| IBIS file imxrt500_ewlb249_v1_3.ibs generated by Viper version: 2020.03.16
| This model valid for
| Part Numbers:   Temperature Range:   Package:
| MIMXRT533SFFOC/MRT533SFFOC   -20C~70C   FOWLP249
| MIMXRT533SFFOCR/MRT533SFFOC   -20C~70C   FOWLP249
| MIMXRT555SFFOC/MRT555SFFOC   -20C~70C   FOWLP249
| MIMXRT555SFFOCR/MRT555SFFOC   -20C~70C   FOWLP249
| MIMXRT595SFFOC/MRT595SFFOC   -20C~70C   FOWLP249
| MIMXRT595SFFOCR/MRT595SFFOC   -20C~70C   FOWLP249
[IBIS Ver]   5.0
[Comment Char]   |_char
[File Name]   imxrt500_ewlb249_v1_3.ibs
[File Rev]   1.2
[Date]   Wed Jan 20 13:06:18 2021
[Source]   NXP Viper 2020.03.16
[Notes]
   Warning 'pullup_ref' Exceeds 15 characters: MIPI_DSI_VDDHA18 was cut to MIPI_DSI_VDDHA1
   Warning 'pullup_ref' Exceeds 15 characters: MIPI_DSI_VDDA_CAP was cut to MIPI_DSI_VDDA_C
[Disclaimer] IMPORTANT NOTICE
  This information is provided on an AS IS basis and without warranty.
  IN NO EVENT SHALL NXP BE LIABLE FOR INCIDENTAL OR CONSEQUENTIAL
  DAMAGES ARISING FROM USE OF THIS INFORMATION. THIS DISCLAIMER OF
  WARRANTY EXTENDS TO THE USER OF THE INFORMATION, AND TO THEIR CUSTOMERS
  OR USERS OF PRODUCTS  AND IS IN LIEU OF ALL WARRANTIES WHETHER EXPRESS,
  IMPLIED, OR STATUTORY, INCLUDING IMPLIED WARRANTIES OF MERCHANTABILITY
  OR FITNESS FOR PARTICULAR PURPOSE.
  NXP does not represent or warrant that the information furnished
  hereunder is free of infringement of any third party patents,
  copyrights, trade secrets, or other intellectual property rights.
  NXP does not represent or warrant that the information is free of
  defect, or that it meets any particular standard, requirements or need
  of the user of the infomation or their customers.
  NXP reserves the right to change the information in this file
  without notice.
   http://www.nxp.com
[Copyright]   (C) Copyright NXP 2004 - 2021, All Rights Reserved.
|   BGA249
[Component]   BGA249
[Manufacturer]   NXP
[Package]
| variable   typ   min   max
R_pkg   0.15592   0.019296   0.4
L_pkg   9.605e-10   9.912e-11   2.758e-09
C_pkg   2.985e-13   9.631e-14   7.183e-13
[Pin] signal_name   model_name   R_pin   L_pin   C_pin
A1   GND   GND   NA   NA   NA
A2   XTALIN32KHZ   POWER   0.323   1.330e-09 4.451e-13
A4   XTALOUTSYS   POWER   0.23297   1.096e-09 4.846e-13
A6   PIO3_12   sd_mmc   0.14311   1.180e-09 3.826e-13
A8   PIO3_8   sd_mmc   0.12255   1.038e-09 3.823e-13
A10   PIO1_0   gpio   0.13766   1.041e-09 3.877e-13
A12   PIO0_28   gpio   0.16732   1.175e-09 4.245e-13
A14   PIO0_21   gpio   0.22629   1.768e-09 4.336e-13
A16   PIO0_16   gpio   0.23815   1.841e-09 4.605e-13
A17   GND   GND   NA   NA   NA
B1   MIPI_DSI_D0P   mipi   0.39132   1.963e-09 5.675e-13
B2   VDD_AO18   POWER   NA   NA   NA
B3   XTALOUT32KHZ   POWER   0.28473   1.432e-09 4.486e-13
B4   XTALINSYS   POWER   0.21088   9.995e-10 3.804e-13
B6   PIO3_18   sd_mmc   0.21102   1.406e-09 4.998e-13
B7   PIO3_13   sd_mmc   0.065009  4.534e-10 2.633e-13
B8   PIO3_9   sd_mmc   0.067056  5.910e-10 1.144e-13
B10   PIO2_29   gpio   0.13988   1.054e-09 2.088e-13
B11   PIO0_29   gpio   0.1449   1.036e-09 2.635e-13
B12   PIO0_14   gpio   0.21245   1.508e-09 4.307e-13
B14   PIO0_22   gpio   0.19354   1.505e-09 1.663e-13
B15   PIO0_15   gpio   0.19156   1.473e-09 2.499e-13
B16   PIO0_18   gpio   0.21271   1.627e-09 3.644e-13
B17   PIO0_17   gpio   0.2616   1.981e-09 4.581e-13
C2   MIPI_DSI_D0N   mipi   0.37397   1.899e-09 3.667e-13
C3   GND   GND   NA   NA   NA
C4   RESETN   gpio   0.13559   6.757e-10 3.401e-13
C5   LDO_ENABLE   gpio   0.032784  2.190e-10 2.165e-13
C6   PIO3_19   gpio   0.055897  5.682e-10 1.332e-13
C7   GND   GND   NA   NA   NA
C8   PIO3_10   sd_mmc   0.058396  5.217e-10 1.117e-13
C9   PIO3_16   sd_mmc   0.12717   1.005e-09 1.378e-13
C10   PIO3_11   sd_mmc   0.19256   1.616e-09 1.355e-13
C11   GND   GND   NA   NA   NA
C12   PIO0_25   gpio   0.12364   1.045e-09 1.356e-13
C13   PIO0_23   gpio   0.16274   1.396e-09 1.592e-13
C14   PIO2_31   gpio   0.16973   9.241e-10 3.844e-13
C15   GND   GND   NA   NA   NA
C16   PIO3_2   gpio   0.18067   1.120e-09 4.565e-13
D1   MIPI_DSI_CLKN   mipi   0.30826   1.261e-09 5.228e-13
D2   MIPI_DSI_CLKP   mipi   0.29277   1.248e-09 3.770e-13
D3   PMIC_MODE0   reset   0.085788  7.054e-10 2.084e-13
D4   VDDEAO   POWER   NA   NA   NA
D5   PMIC_IRQ   gpio   0.019296  9.912e-11 1.330e-13
D6   PIO3_20   gpio   0.12395   8.467e-10 1.799e-13
D7   VSS_ANA   GND   NA   NA   NA
D8   PIO3_17   sd_mmc   0.059128  2.748e-10 1.732e-13
D9   PIO3_14   sd_mmc   0.047493  2.375e-10 1.631e-13
D10   PIO2_30   gpio   0.069171  3.220e-10 1.808e-13
D11   VSS_ADC_ANA   GND   NA   NA   NA
D12   PIO0_31   gpio   0.21896   1.731e-09 2.097e-13
D13   PIO0_24   gpio   0.15029   1.266e-09 1.559e-13
D14   PIO0_30   gpio   0.10947   5.921e-10 2.238e-13
D15   PIO3_3   gpio   0.13521   8.908e-10 1.680e-13
D16   PIO3_1   gpio   0.11241   8.008e-10 2.775e-13
D17   PIO2_15   gpio   0.15691   1.163e-09 4.295e-13
E3   MIPI_DSI_D1P   mipi   0.22048   8.959e-10 4.982e-13
E4   PMIC_MODE1   reset   0.077495  3.186e-10 1.888e-13
E5   PIO3_21   gpio   0.24735   1.577e-09 3.754e-13
E6   VDD_PLL18   POWER   NA   NA   NA
E7   GND   GND   NA   NA   NA
E8   VDD_FUSE18   POWER   NA   NA   NA
E9   VDDE1   POWER   NA   NA   NA
E10   PIO3_15   sd_mmc   0.12196   5.270e-10 2.435e-13
E11   GND   GND   NA   NA   NA
E12   VDD33_ADC_ANA   POWER   NA   NA   NA
E13   PIO4_18   gpio   0.07626   3.382e-10 1.901e-13
E14   PIO0_12   gpio   0.022368  1.796e-10 1.296e-13
E15   PIO2_14   gpio   0.081977  7.304e-10 1.096e-13
F1   PIO4_14   sd_mmc   0.25944   1.688e-09 5.184e-13
F2   PIO4_17   sd_mmc   0.25835   1.776e-09 3.608e-13
F3   MIPI_DSI_D1N   mipi   0.21045   9.219e-10 3.502e-13
F4   MIPI_DSI_VSS   GND   NA   NA   NA
F5   MIPI_DSI_VDDA_CAP   POWER   NA   NA   NA
F6   VDDE4   POWER   NA   NA   NA
F7   VDDE4   POWER   NA   NA   NA
F8   MIPI_DSI_VDDHA18   POWER   NA   NA   NA
F9   VDDE1   POWER   NA   NA   NA
F10   VDDE1   POWER   NA   NA   NA
F11   VDDE1   POWER   NA   NA   NA
F12   VREFH_ANA18   POWER   NA   NA   NA
F13   PIO0_19   gpio   0.097275  4.356e-10 2.152e-13
F14   PIO0_0   gpio   0.088128  3.411e-10 1.672e-13
F15   PIO0_13   gpio   0.07821   6.497e-10 1.711e-13
F16   PIO0_5   gpio   0.081289  5.963e-10 2.780e-13
F17   PIO0_6   gpio   0.13882   1.098e-09 3.874e-13
G2   PIO4_13   sd_mmc   0.22197   1.542e-09 4.236e-13
G3   GND   GND   NA   NA   NA
G4   GND   GND   NA   NA   NA
G5   GND   GND   NA   NA   NA
G6   VDD1V8   POWER   NA   NA   NA
G7   GND   GND   NA   NA   NA
G8   GND   GND   NA   NA   NA
G9   VDDCORE_CAP   POWER   NA   NA   NA
G10   GND   GND   NA   NA   NA
G11   GND   GND   NA   NA   NA
G12   VREFL_ANA   POWER   NA   NA   NA
G13   GND   GND   NA   NA   NA
G14   GND   GND   NA   NA   NA
G15   GND   GND   NA   NA   NA
G16   PIO0_1   gpio   0.10247   4.579e-10 3.732e-13
H1   PIO4_12   sd_mmc   0.13261   1.127e-09 1.525e-13
H2   PIO4_11   sd_mmc   0.084302  6.153e-10 2.604e-13
H3   PIO4_16   sd_mmc   0.11951   1.103e-09 1.622e-13
H4   PIO5_16   sd_mmc   0.062756  3.311e-10 1.766e-13
H5   PIO5_15   sd_mmc   0.072627  3.073e-10 1.838e-13
H6   VDD18_IOREF_1   POWER   NA   NA   NA
H7   VDD1V8_DRV   POWER   NA   NA   NA
H8   VDDCORE_CAP   POWER   NA   NA   NA
H9   VDDCORE_CAP   POWER   NA   NA   NA
H10   VDDCORE_CAP   POWER   NA   NA   NA
H11   GND   GND   NA   NA   NA
H12   PIO0_8   gpio   0.12057   4.423e-10 2.342e-13
H13   VDD18_ADC_ANA   POWER   NA   NA   NA
H14   PIO0_4   gpio   0.047831  2.176e-10 1.585e-13
H15   PIO0_3   gpio   0.058566  4.883e-10 1.263e-13
H16   PIO0_2   gpio   0.092167  5.766e-10 3.745e-13
H17   PIO0_9   gpio   0.14943   8.879e-10 4.225e-13
J3   PIO5_17   sd_mmc   0.038017  3.866e-10 9.631e-14
J4   PIO5_18   sd_mmc   0.073931  3.262e-10 1.803e-13
J5   VDDE1   POWER   NA   NA   NA
J6   VDDE1   POWER   NA   NA   NA
J7   VDD1V8_DRV   POWER   NA   NA   NA
J8   MIPI_DSI_VDD11   POWER   NA   NA   NA
J9   VDDCORE_CAP   POWER   NA   NA   NA
J10   VDDCORE_CAP   POWER   NA   NA   NA
J11   VDDCORE_CAP   POWER   NA   NA   NA
J12   VDDE0   POWER   NA   NA   NA
J13   VDDE0   POWER   NA   NA   NA
J14   VDD18_IOREF_0   POWER   NA   NA   NA
J15   PIO0_7   gpio   0.062602  5.461e-10 1.030e-13
K1   PIO1_4   gpio   0.12726   1.026e-09 4.289e-13
K2   PIO1_3   gpio   0.064288  5.590e-10 3.224e-13
K3   PIO4_15   sd_mmc   0.052393  4.047e-10 1.440e-13
K4   PMIC_I2C_SCL   gpio   0.041685  2.210e-10 1.504e-13
K5   VDD_USB33   POWER   NA   NA   NA
K6   PMIC_I2C_SDA   gpio   0.13049   4.317e-10 3.502e-13
K7   GND   GND   NA   NA   NA
K8   VDDCORE_CAP   POWER   NA   NA   NA
K9   VDDCORE_CAP   POWER   NA   NA   NA
K10   VDDCORE_CAP   POWER   NA   NA   NA
K11   GND   GND   NA   NA   NA
K12   VDDE0   POWER   NA   NA   NA
K13   PIO1_11   gpio   0.073705  2.916e-10 3.894e-13
K14   PIO1_12   gpio   0.050827  2.077e-10 1.709e-13
K15   PIO0_11   gpio   0.061973  4.783e-10 2.714e-13
K16   PIO0_10   gpio   0.12779   7.528e-10 3.663e-13
K17   PIO1_13   gpio   0.13572   9.556e-10 4.001e-13
L2   PIO1_5   gpio   0.075752  5.651e-10 2.551e-13
L3   GND   GND   NA   NA   NA
L4   GND   GND   NA   NA   NA
L5   GND   GND   NA   NA   NA
L6   GND   GND   NA   NA   NA
L7   GND   GND   NA   NA   NA
L8   GND   GND   NA   NA   NA
L9   VDDCORE_CAP   POWER   NA   NA   NA
L10   GND   GND   NA   NA   NA
L11   GND   GND   NA   NA   NA
L12   GND   GND   NA   NA   NA
L13   GND   GND   NA   NA   NA
L14   GND   GND   NA   NA   NA
L15   GND   GND   NA   NA   NA
L16   PIO1_14   gpio   0.086255  5.497e-10 3.068e-13
M1   PIO1_7   gpio   0.19046   1.385e-09 5.761e-13
M2   PIO2_25   gpio   0.13329   1.029e-09 3.646e-13
M3   PIO2_27   gpio   0.082138  2.978e-10 1.572e-13
M4   PIO2_26   gpio   0.085997  3.288e-10 1.757e-13
M5   PIO1_10   gpio   0.079525  3.383e-10 1.749e-13
M6   VDD_USB18   POWER   NA   NA   NA
M7   GND   GND   NA   NA   NA
M8   VDDE3   POWER   NA   NA   NA
M9   PIO5_1   gpiohv   0.17413   6.089e-10 4.540e-13
M10   VDDE0   POWER   NA   NA   NA
M11   GND   GND   NA   NA   NA
M12   VDDE0   POWER   NA   NA   NA
M13   PIO3_29   gpio   0.20028   7.768e-10 3.196e-13
M14   PIO4_3   gpio   0.072546  3.197e-10 1.837e-13
M15   PIO4_1   gpio   0.11381   8.533e-10 2.816e-13
M16   PIO1_15   gpio   0.16285   5.641e-10 4.457e-13
M17   PIO4_2   gpio   0.15728   1.014e-09 4.269e-13
N3   PIO2_24   gpio   0.11438   5.537e-10 1.723e-13
N4   PIO1_6   gpio   0.062866  3.020e-10 1.892e-13
N5   PIO2_10   gpio   0.073482  3.155e-10 1.841e-13
N6   VDDE2   POWER   NA   NA   NA
N7   GND   GND   NA   NA   NA
N8   PIO4_30   gpiohv   0.11743   4.531e-10 2.355e-13
N9   VDDE3   POWER   NA   NA   NA
N10   PIO4_31   gpiohv   0.17786   6.915e-10 3.013e-13
N11   GND   GND   NA   NA   NA
N12   PIO1_24   sd_mmc   0.27515   9.660e-10 3.982e-13
N13   PIO3_28   gpio   0.18841   6.032e-10 2.830e-13
N14   PIO3_27   gpio   0.22419   7.513e-10 3.286e-13
N15   PIO4_0   gpio   0.050214  4.488e-10 9.853e-14
P1   PIO2_28   gpio   0.23077   8.666e-10 4.913e-13
P2   PIO5_4   gpio   0.18895   8.361e-10 2.819e-13
P3   PIO5_8   gpio   0.16805   5.890e-10 3.961e-13
P4   PIO2_7   sd_mmc   0.046303  2.501e-10 1.483e-13
P5   PIO2_5   sd_mmc   0.036306  2.135e-10 1.439e-13
P6   PIO2_4   sd_mmc   0.069851  3.058e-10 1.856e-13
P7   VDDE2   POWER   NA   NA   NA
P8   PIO4_29   gpiohv   0.074088  3.644e-10 1.958e-13
P9   PIO4_27   gpiohv   0.15417   6.758e-10 2.585e-13
P10   PIO4_21   gpiohv   0.1396   5.865e-10 2.562e-13
P11   GND   GND   NA   NA   NA
P12   PIO5_0   gpiohv   0.31252   2.244e-09 3.349e-13
P13   PIO1_27   sd_mmc   0.23594   1.837e-09 2.443e-13
P14   PIO1_26   sd_mmc   0.30392   1.154e-09 4.566e-13
P15   PIO4_6   gpio   0.061648  4.596e-10 1.742e-13
P16   PIO4_5   gpio   0.20809   1.756e-09 4.205e-13
P17   PIO4_4   gpio   0.1891   1.545e-09 3.954e-13
R2   PIO2_11   gpio   0.12089   8.885e-10 1.990e-13
R3   GND   GND   NA   NA   NA
R4   PIO2_6   sd_mmc   0.067012  6.136e-10 9.890e-14
R5   PIO1_30   sd_mmc   0.068108  3.900e-10 1.962e-13
R6   PIO1_31   sd_mmc   0.056674  4.622e-10 1.939e-13
R7   GND   GND   NA   NA   NA
R8   PIO4_20   gpiohv   0.057557  5.489e-10 1.040e-13
R9   PIO5_2   gpiohv   0.091773  6.332e-10 1.818e-13
R10   PIO5_3   gpiohv   0.13625   8.187e-10 2.283e-13
R11   GND   GND   NA   NA   NA
R12   PIO1_23   sd_mmc   0.30732   1.355e-09 4.114e-13
R13   PIO1_22   sd_mmc   0.2423   1.910e-09 2.292e-13
R14   PIO1_25   sd_mmc   0.3338   2.453e-09 2.757e-13
R15   GND   GND   NA   NA   NA
R16   PIO3_25   gpio   0.27408   1.989e-09 2.302e-13
T1   USB0_DM   usbdpdm   0.35276   1.717e-09 5.051e-13
T2   USB0_VBUS_DETECT   POWER   0.26142   1.418e-09 4.000e-13
T3   PIO2_9   gpio   0.092275  7.827e-10 3.446e-13
T4   PIO2_1   sd_mmc   0.083664  7.075e-10 3.423e-13
T6   PIO2_8   sd_mmc   0.11338   1.080e-09 2.706e-13
T7   PIO2_2   sd_mmc   0.11182   1.072e-09 2.535e-13
T8   PIO4_23   gpiohv   0.087906  6.854e-10 2.884e-13
T10   PIO4_24   gpiohv   0.13973   9.951e-10 2.208e-13
T11   PIO4_25   gpiohv   0.25374   1.734e-09 2.601e-13
T12   PIO4_26   gpiohv   0.26837   1.817e-09 2.982e-13
T14   PIO1_21   sd_mmc   0.36032   1.841e-09 4.475e-13
T15   PIO1_20   sd_mmc   0.38127   1.797e-09 4.826e-13
T16   PIO3_26   gpio   0.28345   1.995e-09 4.672e-13
T17   PIO1_18   sd_mmc   0.394   2.758e-09 5.564e-13
U1   GND   GND   NA   NA   NA
U2   USB0_DP   usbdpdm   0.33611   1.796e-09 4.815e-13
U4   PIO2_0   sd_mmc   0.18718   1.342e-09 4.224e-13
U6   PIO2_3   sd_mmc   0.17593   1.363e-09 5.005e-13
U8   PIO4_28   gpiohv   0.14778   1.113e-09 3.807e-13
U10   PIO4_22   gpiohv   0.19253   1.246e-09 4.489e-13
U12   PIO1_29   sd_mmc   0.28287   1.985e-09 5.064e-13
U14   PIO1_28   sd_mmc   0.29826   2.149e-09 5.288e-13
U16   PIO1_19   sd_mmc   0.4   2.303e-09 7.183e-13
U17   GND   GND   NA   NA   NA
[Pin Mapping]   pulldown_ref   pullup_ref
A1   GND   NC
A2   NC   VDDEAO
A4   NC   VDD_FUSE18
A6   GND   VDDE4
A8   GND   VDDE4
A10   GND   VDDE1
A12   GND   VDDE1
A14   GND   VDDE1
A16   GND   VDDE1
A17   GND   NC
B1   GND   MIPI_DSI_VDDHA1
B2   NC   VDD_AO18
B3   NC   VDDEAO
B4   NC   VDD_FUSE18
B6   GND   VDDE4
B7   GND   VDDE4
B8   GND   VDDE4
B10   GND   VDDE1
B11   GND   VDDE1
B12   GND   VDDE1
B14   GND   VDDE1
B15   GND   VDDE1
B16   GND   VDDE1
B17   GND   VDDE1
C2   GND   MIPI_DSI_VDDHA1
C3   GND   NC
C4   GND   VDDEAO
C5   GND   VDDEAO
C6   GND   VDDE4
C7   GND   NC
C8   GND   VDDE4
C9   GND   VDDE4
C10   GND   VDDE4
C11   GND   NC
C12   GND   VDDE1
C13   GND   VDDE1
C14   GND   VDDE1
C15   GND   NC
C16   GND   VDDE1
D1   GND   MIPI_DSI_VDDHA1
D2   GND   MIPI_DSI_VDDHA1
D3   GND   VDDEAO
D4   NC   VDDEAO
D5   GND   VDDEAO
D6   GND   VDDE4
D7   GND   NC
D8   GND   VDDE4
D9   GND   VDDE4
D10   GND   VDDE1
D11   VSS_ADC_ANA   NC
D12   GND   VDDE1
D13   GND   VDDE1
D14   GND   VDDE1
D15   GND   VDDE1
D16   GND   VDDE1
D17   GND   VDDE0
E3   GND   MIPI_DSI_VDDHA1
E4   GND   VDDEAO
E5   GND   VDDE4
E6   NC   VDD_PLL18
E7   GND   NC
E8   NC   VDD_FUSE18
E9   NC   VDDE1
E10   GND   VDDE4
E11   GND   NC
E12   NC   VDD33_ADC_ANA
E13   GND   VDDE1
E14   GND   VDDE0
E15   GND   VDDE0
F1   GND   VDDE1
F2   GND   VDDE1
F3   GND   MIPI_DSI_VDDHA1
F4   GND   NC
F5   NC   MIPI_DSI_VDDA_C
F6   NC   VDDE4
F7   NC   VDDE4
F8   NC   MIPI_DSI_VDDHA1
F9   NC   VDDE1
F10   NC   VDDE1
F11   NC   VDDE1
F12   NC   VDD18_ADC_ANA
F13   GND   VDDE1
F14   GND   VDDE0
F15   GND   VDDE0
F16   GND   VDDE0
F17   GND   VDDE0
G2   GND   VDDE1
G3   GND   NC
G4   GND   NC
G5   GND   NC
G6   NC   VDDEAO
G7   GND   NC
G8   GND   NC
G9   NC   VDDE0
G10   GND   NC
G11   GND   NC
G12   NC   VDD18_ADC_ANA
G13   GND   NC
G14   GND   NC
G15   GND   NC
G16   GND   VDDE0
H1   GND   VDDE1
H2   GND   VDDE1
H3   GND   VDDE1
H4   GND   VDDE1
H5   GND   VDDE1
H6   NC   VDDE1
H7   NC   VDDEAO
H8   NC   VDDE0
H9   NC   VDDE0
H10   NC   VDDE0
H11   GND   NC
H12   GND   VDDE0
H13   NC   VDD33_ADC_ANA
H14   GND   VDDE0
H15   GND   VDDE0
H16   GND   VDDE0
H17   GND   VDDE0
J3   GND   VDDE1
J4   GND   VDDE1
J5   NC   VDDE1
J6   NC   VDDE1
J7   NC   VDDEAO
J8   NC   MIPI_DSI_VDD11
J9   NC   VDDE0
J10   NC   VDDE0
J11   NC   VDDE0
J12   NC   VDDE0
J13   NC   VDDE0
J14   NC   VDDE0
J15   GND   VDDE0
K1   GND   VDDE1
K2   GND   VDDE1
K3   GND   VDDE1
K4   GND   VDDE1
K5   NC   VDD_USB33
K6   GND   VDDE1
K7   GND   NC
K8   NC   VDDE0
K9   NC   VDDE0
K10   NC   VDDE0
K11   GND   NC
K12   NC   VDDE0
K13   GND   VDDE0
K14   GND   VDDE0
K15   GND   VDDE0
K16   GND   VDDE0
K17   GND   VDDE0
L2   GND   VDDE1
L3   GND   NC
L4   GND   NC
L5   GND   NC
L6   GND   NC
L7   GND   NC
L8   GND   NC
L9   NC   VDDE0
L10   GND   NC
L11   GND   NC
L12   GND   NC
L13   GND   NC
L14   GND   NC
L15   GND   NC
L16   GND   VDDE0
M1   GND   VDDE1
M2   GND   VDDE1
M3   GND   VDDE1
M4   GND   VDDE1
M5   GND   VDDE1
M6   NC   VDD_USB33
M7   GND   NC
M8   NC   VDDE3
M9   GND   VDDE3
M10   NC   VDDE0
M11   GND   NC
M12   NC   VDDE0
M13   GND   VDDE0
M14   GND   VDDE0
M15   GND   VDDE0
M16   GND   VDDE0
M17   GND   VDDE0
N3   GND   VDDE1
N4   GND   VDDE1
N5   GND   VDDE2
N6   NC   VDDE2
N7   GND   NC
N8   GND   VDDE3
N9   NC   VDDE3
N10   GND   VDDE3
N11   GND   NC
N12   GND   VDDE0
N13   GND   VDDE0
N14   GND   VDDE0
N15   GND   VDDE0
P1   GND   VDDE1
P2   GND   VDDE1
P3   GND   VDDE1
P4   GND   VDDE2
P5   GND   VDDE2
P6   GND   VDDE2
P7   NC   VDDE2
P8   GND   VDDE3
P9   GND   VDDE3
P10   GND   VDDE3
P11   GND   NC
P12   GND   VDDE3
P13   GND   VDDE0
P14   GND   VDDE0
P15   GND   VDDE0
P16   GND   VDDE0
P17   GND   VDDE0
R2   GND   VDDE2
R3   GND   NC
R4   GND   VDDE2
R5   GND   VDDE2
R6   GND   VDDE2
R7   GND   NC
R8   GND   VDDE3
R9   GND   VDDE3
R10   GND   VDDE3
R11   GND   NC
R12   GND   VDDE0
R13   GND   VDDE0
R14   GND   VDDE0
R15   GND   NC
R16   GND   VDDE0
T1   GND   VDD_USB33
T2   NC   VDD_USB33
T3   GND   VDDE2
T4   GND   VDDE2
T6   GND   VDDE2
T7   GND   VDDE2
T8   GND   VDDE3
T10   GND   VDDE3
T11   GND   VDDE3
T12   GND   VDDE3
T14   GND   VDDE0
T15   GND   VDDE0
T16   GND   VDDE0
T17   GND   VDDE0
U1   GND   NC
U2   GND   VDD_USB33
U4   GND   VDDE2
U6   GND   VDDE2
U8   GND   VDDE3
U10   GND   VDDE3
U12   GND   VDDE0
U14   GND   VDDE0
U16   GND   VDDE0
U17   GND   NC
[Diff Pin]  inv_pin  vdiff  tdelay_typ tdelay_min tdelay_max
B1   C2   NA   NA   NA   NA
D2   D1   NA   NA   NA   NA
E3   F3   NA   NA   NA   NA
T1   U2   NA   NA   NA   NA
|*   Model Selector   *
[Model Selector] gpio
io_obe1dse0sre0_lr   5mA current driving capability, w/o slew rate (Low Range Typ: 1.80V, Min: 1.71V, Max: 1.98V)
io_obe1dse0sre1_lr   5mA current driving capability, with slew rate (Low Range Typ: 1.80V, Min: 1.71V, Max: 1.98V)
io_obe1dse1sre0_lr   10mA current driving capability, w/o slew rate (Low Range Typ: 1.80V, Min: 1.71V, Max: 1.98V)
io_obe1dse1sre1_lr   10mA current driving capability, with slew rate (Low Range Typ: 1.80V, Min: 1.71V, Max: 1.98V)
[Model Selector] gpiohv
io_obe1dse0sre0_hr   5mA current driving capability, w/o slew rate (High Range Typ: 3.30V, Min: 3.00V, Max: 3.60V)
io_obe1dse0sre0_lr   5mA current driving capability, w/o slew rate (Low Range Typ: 1.80V, Min: 1.71V, Max: 1.98V)
io_obe1dse0sre0_nr   5mA current driving capability, w/o slew rate (Cont. Range Typ: 3.30V, Min: 2.70V, Max: 3.60V)
io_obe1dse0sre1_hr   5mA current driving capability, with slew rate (High Range Typ: 3.30V, Min: 3.00V, Max: 3.60V)
io_obe1dse0sre1_lr   5mA current driving capability, with slew rate (Low Range Typ: 1.80V, Min: 1.71V, Max: 1.98V)
io_obe1dse0sre1_nr   5mA current driving capability, with slew rate (Cont. Range Typ: 3.30V, Min: 2.70V, Max: 3.60V)
io_obe1dse1sre0_hr   10mA current driving capability, w/o slew rate (High Range Typ: 3.30V, Min: 3.00V, Max: 3.60V)
io_obe1dse1sre0_lr   10mA current driving capability, w/o slew rate (Low Range Typ: 1.80V, Min: 1.71V, Max: 1.98V)
io_obe1dse1sre0_nr   10mA current driving capability, w/o slew rate (Cont. Range Typ: 3.30V, Min: 2.70V, Max: 3.60V)
io_obe1dse1sre1_hr   10mA current driving capability, with slew rate (High Range Typ: 3.30V, Min: 3.00V, Max: 3.60V)
io_obe1dse1sre1_lr   10mA current driving capability, with slew rate (Low Range Typ: 1.80V, Min: 1.71V, Max: 1.98V)
io_obe1dse1sre1_nr   10mA current driving capability, with slew rate (Cont. Range Typ: 3.30V, Min: 2.70V, Max: 3.60V)
[Model Selector] mipi
MIPI_HS   MIPI DSI High Speed Mode
MIPI_LP   MIPI DSI Low Power Mode
[Model Selector] reset
io_rst_obe1dse0sre0_lr   5mA current driving capability, w/o slew rate (Low Range Typ: 1.80V, Min: 1.71V, Max: 1.98V)
io_rst_obe1dse0sre1_lr   5mA current driving capability, with slew rate (Low Range Typ: 1.80V, Min: 1.71V, Max: 1.98V)
io_rst_obe1dse1sre0_lr   10mA current driving capability, w/o slew rate (Low Range Typ: 1.80V, Min: 1.71V, Max: 1.98V)
io_rst_obe1dse1sre1_lr   10mA current driving capability, with slew rate (Low Range Typ: 1.80V, Min: 1.71V, Max: 1.98V)
[Model Selector] sd_mmc
BDPROGSCARUDQP_SDMMC_3V3SF_00_MMC   PSW=0 PDRV=0 MODE=1V8 MMC
BDPROGSCARUDQP_SDMMC_3V3SF_00_SD   PSW=0 PDRV=0 MODE=1V8 SD
BDPROGSCARUDQP_SDMMC_3V3SF_01_MMC   PSW=0 PDRV=1 MODE=1V8 MMC
BDPROGSCARUDQP_SDMMC_3V3SF_01_SD   PSW=0 PDRV=1 MODE=1V8 SD
[Model Selector] usbdpdm
FS_driver   Full Speed USB driver
HS_driver   High Speed USB driver
LS_driver   Low Speed USB driver
fs_device_dm_input   Full Speed Device dm Input
fs_device_dp_input   Full Speed Device dp Input
fs_host_input   Full Speed Host Input
hs_input   High Speed USB Input
ls_host_input   Low  Speed Host Input
| End [Component] BGA249
| Models and submodels in the file (30): BDPROGSCARUDQP_SDMMC_3V3SF_00_MMC (I/O), BDPROGSCARUDQP_SDMMC_3V3SF_00_SD (I/O), BDPROGSCARUDQP_SDMMC_3V3SF_01_MMC (I/O), BDPROGSCARUDQP_SDMMC_3V3SF_01_SD (I/O), FS_driver (Output), HS_driver (Output), LS_driver (Output), MIPI_HS (Output), MIPI_LP (I/O), fs_device_dm_input (Input), fs_device_dp_input (Input), fs_host_input (Input), hs_input (Input), io_obe1dse0sre0_hr (I/O), io_obe1dse0sre0_lr (I/O), io_obe1dse0sre0_nr (I/O), io_obe1dse0sre1_hr (I/O), io_obe1dse0sre1_lr (I/O), io_obe1dse0sre1_nr (I/O), io_obe1dse1sre0_hr (I/O), io_obe1dse1sre0_lr (I/O), io_obe1dse1sre0_nr (I/O), io_obe1dse1sre1_hr (I/O), io_obe1dse1sre1_lr (I/O), io_obe1dse1sre1_nr (I/O), io_rst_obe1dse0sre0_lr (I/O), io_rst_obe1dse0sre1_lr (I/O), io_rst_obe1dse1sre0_lr (I/O), io_rst_obe1dse1sre1_lr (I/O), ls_host_input (Input)
